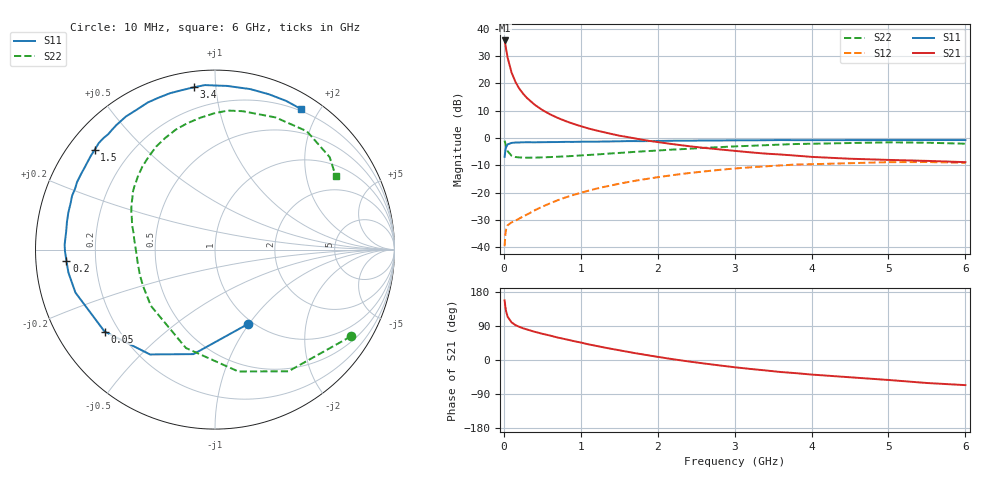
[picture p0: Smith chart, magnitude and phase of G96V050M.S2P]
! SIEMENS Small Signal Semiconductors
! BFG235
! Si NPN RF Bipolar Junction Transistor in SOT223
! VCE = 6 V  IC = 50 mA
! Common Emitter S-Parameters:  July  1994
# GHz  S  MA  R  50
!  f  S11  S21  S12  S22
! GHz  MAG  ANG  MAG  ANG  MAG  ANG  MAG  ANG
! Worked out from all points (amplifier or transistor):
!   40 points, 10 MHz to 6 GHz, reference 50 ohm
!   highest |S21| = 35.7 dB at 10 MHz (marker M1)
!   |S21| within 3 dB of that: start of sweep to 28.57 MHz
!   unconditionally stable (mu >= 1): 516.6 MHz to 1.318 GHz
!   at 200 MHz: K = 0.67, MSG = 23.8 dB, |S12| = -29.5 dB
!   at 1.5 GHz: K = 0.97, MSG = 8.8 dB, |S12| = -16.7 dB
!   at 6 GHz: K = 0.92, MSG = 0.1 dB, |S12| = -9.1 dB
!   S11 on the Smith chart (normalised r, x): 10 MHz: 0.95, -0.99; 50 MHz: 0.15, -0.32; 200 MHz: 0.09, -0.04; 1.5 GHz: 0.08, +0.36; 3.4 GHz: 0.08, +0.87; 6 GHz: 0.18, +1.77
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0.01  0.4532 -65.8  61.03 157.3  0.0105 69.6  0.8988 -32.5
0.02  0.5944 -101.6  50.97 140.1  0.0174 54.7  0.7919 -58.9
0.03  0.6873 -121.8  42.03 127.9  0.0215 44.6  0.6912 -79.2
0.05  0.7661 -143.4  29.24 113.9  0.0254 34.1  0.5716 -106.5
0.1  0.8137 -162.9  15.87 99.4  0.0286 30.6  0.475 -138.8
0.15  0.8268 -171.1  10.71 92.2  0.0306 33.7  0.4492 -153.2
0.2  0.83 -175.6  8.046 87.6  0.0336 37.2  0.4419 -161.4
0.25  0.8359 -179.3  6.487 83.7  0.0367 40.8  0.4375 -166.7
0.3  0.8382 178.1  5.418 80.6  0.0397 44.1  0.4369 -170.9
0.4  0.8353 173.0  4.075 74.5  0.0475 47.9  0.438 -176.7
0.5  0.8393 169.3  3.259 69.2  0.0555 50.9  0.4426 179.0
0.6  0.8427 165.9  2.719 64.5  0.0638 52.3  0.4481 175.4
0.7  0.8449 162.2  2.338 59.3  0.0728 53.3  0.4552 172.1
0.9  0.8501 156.6  1.827 50.3  0.0904 52.6  0.4701 166.5
1.1  0.8571 150.2  1.495 41.3  0.1087 50.8  0.4899 160.9
1.5  0.871 140.4  1.106 25.7  0.1458 44.9  0.534 150.2
2.2  0.8923 123.8  0.772 2.0  0.2099 30.9  0.6151 131.1
3.2  0.9073 101.8  0.548 -23.5  0.2906 7.3  0.7202 102.6
3.4  0.9118 97.5  0.519 -27.5  0.3034 2.2  0.7389 96.4
4.5  0.9156 77.6  0.418 -45.6  0.3464 -24.0  0.81 65.4
5.5  0.9184 64.4  0.382 -60.7  0.3634 -46.5  0.8209 38.9
6  0.9182 58.5  0.362 -66.3  0.3524 -54.9  0.7871 31.3
